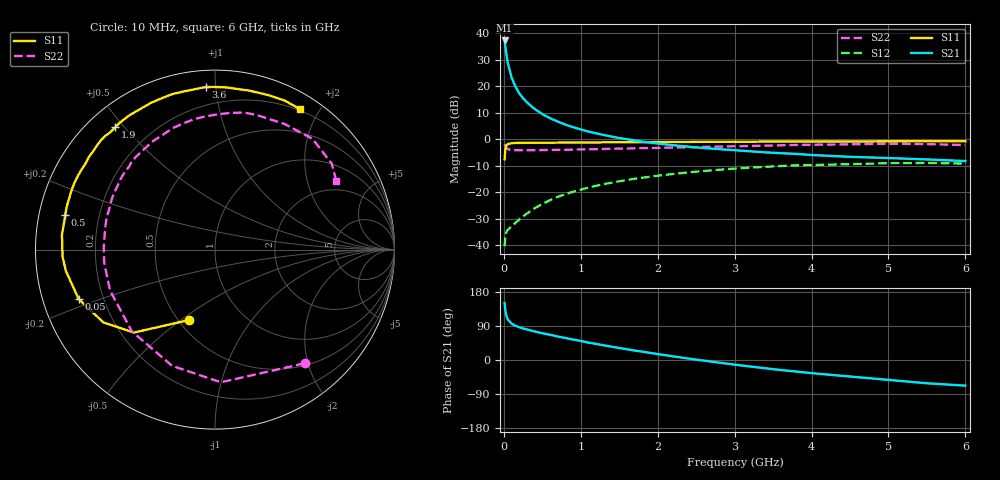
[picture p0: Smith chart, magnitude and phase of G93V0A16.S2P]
! SIEMENS Small Signal Semiconductors
! BFG235
! Si NPN RF Bipolar Junction Transistor in SOT223
! VCE = 3 V  IC = 160 mA
! Common Emitter S-Parameters:  July  1994
# GHz  S  MA  R  50
!  f  S11  S21  S12  S22
! GHz  MAG  ANG  MAG  ANG  MAG  ANG  MAG  ANG
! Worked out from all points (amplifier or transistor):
!   40 points, 10 MHz to 6 GHz, reference 50 ohm
!   highest |S21| = 37.2 dB at 10 MHz (marker M1)
!   |S21| within 3 dB of that: start of sweep to 22.86 MHz
!   unconditionally stable (mu >= 1): 434.5 MHz to 1.528 GHz
!   at 200 MHz: K = 0.82, MSG = 23.8 dB, |S12| = -30.3 dB
!   at 1.5 GHz: K = 1.00, MAG = 7.8 dB, |S12| = -15.9 dB
!   at 6 GHz: K = 0.92, MSG = 0.5 dB, |S12| = -9.2 dB
!   S11 on the Smith chart (normalised r, x): 10 MHz: 0.56, -0.53; 50 MHz: 0.11, -0.17; 500 MHz: 0.08, +0.11; 1.9 GHz: 0.08, +0.47; 3.6 GHz: 0.09, +0.94; 6 GHz: 0.18, +1.76
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0.01  0.4194 -110.5  72.81 150.2  0.0096 59.5  0.8065 -51.8
0.02  0.6456 -134.3  55.55 130.6  0.0145 45.8  0.74 -87.5
0.03  0.7427 -146.9  42.76 119.1  0.0172 38.8  0.6903 -110.3
0.05  0.808 -160.1  28.03 107.3  0.0195 33.0  0.6496 -135.5
0.1  0.8395 -171.9  14.66 96.0  0.0227 37.1  0.6276 -158.7
0.15  0.8503 -177.4  9.831 90.2  0.0263 43.4  0.6195 -168.3
0.2  0.8506 179.7  7.351 86.5  0.0305 48.4  0.6213 -173.7
0.25  0.8526 176.8  5.925 83.2  0.0352 52.5  0.6189 -177.6
0.3  0.8568 174.6  4.944 80.6  0.0396 55.0  0.6201 179.1
0.4  0.8542 170.3  3.725 75.3  0.0498 57.2  0.6194 174.2
0.5  0.8564 166.9  2.975 70.7  0.0601 58.3  0.6226 170.1
0.7  0.8618 160.2  2.15 62.0  0.0817 57.4  0.6298 162.8
0.9  0.8669 154.9  1.686 54.0  0.102 54.5  0.6354 156.5
1.1  0.867 148.6  1.389 45.8  0.1225 50.9  0.6456 150.2
1.4  0.8724 141.2  1.12 35.0  0.1512 44.7  0.6592 141.7
1.9  0.8798 129.2  0.862 18.8  0.1959 33.6  0.6814 127.7
2.2  0.8873 122.7  0.771 9.6  0.2206 26.8  0.6962 119.8
3.2  0.8982 101.4  0.591 -17.1  0.2906 3.5  0.7443 94.0
3.6  0.9075 93.2  0.545 -26.5  0.3115 -6.3  0.7672 83.1
4.5  0.906 77.9  0.465 -43.6  0.3384 -25.7  0.8003 60.9
5.5  0.9164 64.9  0.415 -61.4  0.3562 -47.3  0.8078 36.4
6  0.9152 58.8  0.387 -67.7  0.3463 -55.4  0.7758 29.3
